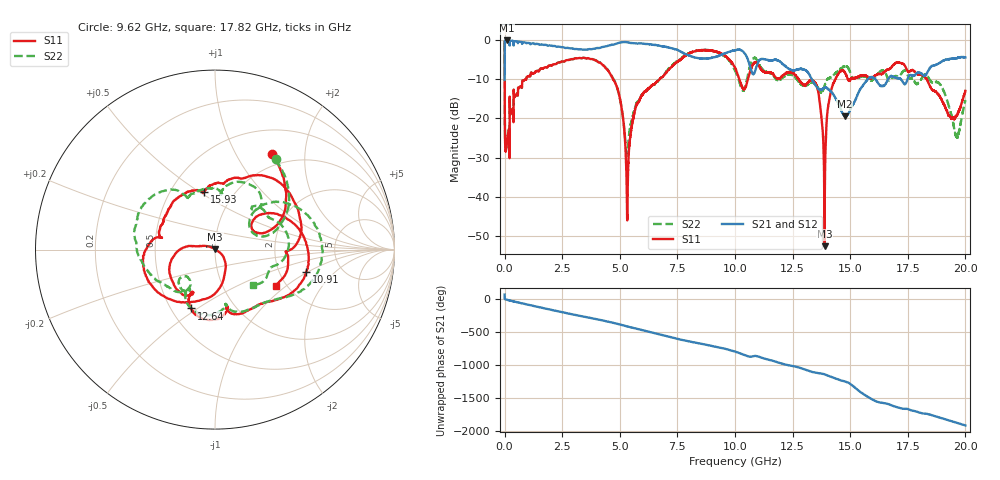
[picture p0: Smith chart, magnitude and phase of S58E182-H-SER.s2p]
!{S58E182}
!Johanson Technology Inc.
!www.johansontechnology.com
!Test Board Conditions:
!Substrate Type  RO4350B
!Substrate Thickness  60 mil
!Substrate Dk  3.66
!TL Type: GCPW
!TL Trace Width  115 mil
!TL Gap  52 mil
!Electrode orientation  Horizontal
!DUT TOPOLOGY	SERIES
!Mounting Pad LxW  55x428 mil
! Created Wed Apr 14 11:25:43 2021
# mhz S ma R 50
! 2 Port Network Data from SP1.SP block
! freq  magS11  angS11  magS21  angS21  magS12  angS12  magS22  angS22
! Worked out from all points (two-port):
!   20001 points, 300 kHz to 20 GHz, reference 50 ohm
!   highest |S21| = -0.02 dB at 86.3 MHz (marker M1); lowest = -19.4 dB at 14.76 GHz (marker M2)
!   |S21| within 3 dB of the highest: 1.148 MHz to 7.678 GHz (7.677 GHz wide, 200 % of centre); 9.706 GHz to 10.38 GHz (672 MHz wide, 6.69 % of centre)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
!   lowest |S11| = -52.7 dB at 13.89 GHz (marker M3), VSWR 1.00, Z = 50.2 + j0.168 ohm
!   |S11| at or under -10 dB: 4.714 GHz to 6.715 GHz (2.001 GHz wide, 35 % of centre); 12.77 GHz to 14.35 GHz (1.586 GHz wide, 11.7 % of centre); 18.32 GHz to end of sweep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
!   |S22| runs from -30.1 to -0.5 dB; largest |S21 - S12| = 0.01
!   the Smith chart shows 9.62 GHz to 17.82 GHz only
!   S11 on the Smith chart (normalised r, x): 9.62 GHz: 0.83, +1.43; 10.91 GHz: 2.83, -0.96; 12.64 GHz: 0.63, -0.47; 15.93 GHz: 0.72, +0.52; 17.82 GHz: 1.75, -0.84
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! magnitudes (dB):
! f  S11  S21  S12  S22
! 300 kHz  -0.5  -10.1  -10.1  -0.5
! 86.3 MHz  -27.0  0.0  0.0  -27.0
! 867.3 MHz  -10.1  -0.5  -0.5  -10.1
! 3.334 GHz  -4.6  -2.3  -2.3  -4.6
! 4.831 GHz  -11.3  -0.9  -0.9  -11.2
! 5.326 GHz  -43.0  -0.5  -0.5  -29.1
! 5.709 GHz  -16.8  -0.7  -0.7  -16.3
! 6.667 GHz  -10.3  -1.3  -1.3  -10.4
! 9.62 GHz  -4.2  -3.2  -3.3  -4.3
! 10 GHz  -7.0  -2.6  -2.6  -7.7
! 10.91 GHz  -5.6  -7.1  -7.1  -4.7
! 12.64 GHz  -9.0  -7.6  -7.5  -9.5
! 13.33 GHz  -10.2  -10.0  -9.9  -10.8
! 13.89 GHz  -52.7  -12.1  -11.9  -11.6
! 14.18 GHz  -12.6  -13.3  -13.2  -9.3
! 14.76 GHz  -8.2  -19.4  -19.4  -6.7
! 15.93 GHz  -9.7  -9.4  -9.3  -10.3
! 16.67 GHz  -7.5  -9.7  -9.7  -10.3
! 17.82 GHz  -8.1  -8.8  -8.8  -10.8
! 18.91 GHz  -14.6  -5.7  -5.7  -11.3
! 19.62 GHz  -19.3  -4.5  -4.5  -24.7
! 20 GHz  -12.9  -4.4  -4.2  -15.3
